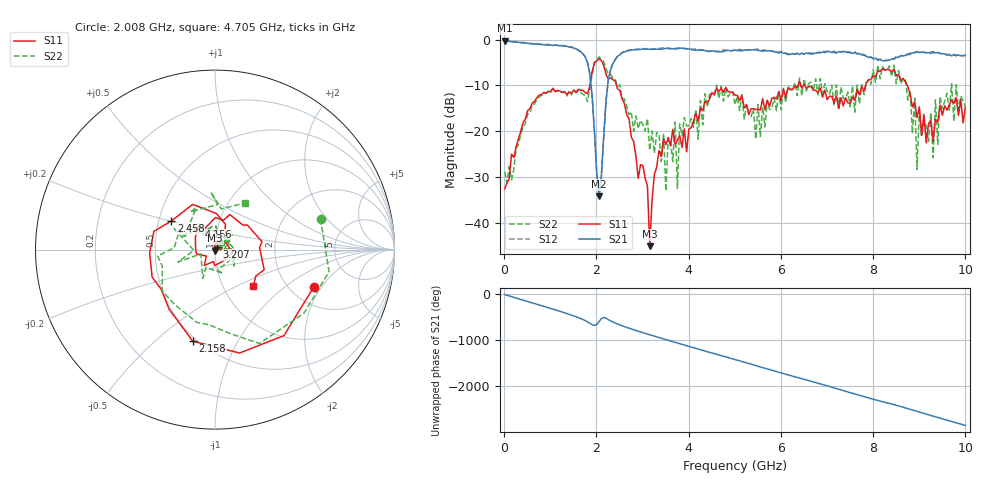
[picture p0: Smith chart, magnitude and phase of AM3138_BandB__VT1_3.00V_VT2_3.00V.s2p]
! Date/Time: Tue, Nov 13, 2018 4:39 PM
! Network Analyzer: Agilent Technologies E8364B Rev: A.07.50.67
! Sweep from 0.010 to 10.000 GHz, 201 Points, Sweep Type: LIN
! Power Supply: 3.001 V, 0.000 A
# Hz S DB R 50
!freq MagS11 AngS11 MagS21 AngS21 MagS12 AngS12 MagS22 AngS22
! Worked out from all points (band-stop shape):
!   201 points, 10 MHz to 10 GHz, reference 50 ohm
!   highest |S21| = -0.23 dB at 10 MHz (marker M1); lowest = -34.1 dB at 2.058 GHz (marker M2)
!   |S21| within 3 dB of the highest: start of sweep to 1.715 GHz; 2.521 GHz to 6.142 GHz (3.621 GHz wide, 83.6 % of centre)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
!   lowest |S11| = -45.0 dB at 3.157 GHz (marker M3), VSWR 1.01, Z = 50 - j0.564 ohm
!   |S11| at or under -10 dB: start of sweep to 1.859 GHz; 2.437 GHz to 6.369 GHz (3.932 GHz wide, 89.3 % of centre); 6.515 GHz to 7.836 GHz (1.321 GHz wide, 18.4 % of centre)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
!   |S22| runs from -33.0 to -3.8 dB; largest |S21 - S12| = 0.029
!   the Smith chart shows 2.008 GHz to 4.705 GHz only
!   S11 on the Smith chart (normalised r, x): 2.008 GHz: 2.64, -1.70; 2.158 GHz: 0.48, -0.67; 2.458 GHz: 0.58, +0.20; 3.207 GHz: 1.02, +0.03; 4.156 GHz: 0.81, +0.21; 4.705 GHz: 1.38, -0.62
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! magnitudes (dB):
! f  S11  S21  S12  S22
! 10 MHz  -32.5  -0.2  -0.2  -28.7
! 1.708 GHz  -11.1  -3.1  -3.0  -11.9
! 2.008 GHz  -4.6  -29.2  -29.0  -4.3
! 2.058 GHz  -4.2  -34.1  -34.3  -3.8
! 2.158 GHz  -5.6  -21.3  -21.3  -4.7
! 2.458 GHz  -10.7  -3.7  -3.6  -10.3
! 3.157 GHz  -45.0  -2.1  -2.1  -24.1
! 3.207 GHz  -34.8  -2.1  -2.1  -19.9
! 3.357 GHz  -24.2  -2.1  -1.9  -20.6
! 3.507 GHz  -22.8  -1.9  -1.9  -33.0
! 3.706 GHz  -22.8  -2.1  -1.9  -17.9
! 3.756 GHz  -21.9  -2.0  -1.9  -32.4
! 3.806 GHz  -20.9  -1.9  -1.8  -18.4
! 4.156 GHz  -16.1  -2.3  -2.1  -15.2
! 4.705 GHz  -10.6  -2.7  -2.5  -10.2
! 5.005 GHz  -12.1  -2.3  -2.2  -14.2
! 6.703 GHz  -11.0  -3.1  -2.9  -11.2
! 8.352 GHz  -6.6  -4.5  -4.4  -5.7
! 8.901 GHz  -13.5  -2.9  -2.8  -12.8
! 8.951 GHz  -17.0  -2.7  -2.6  -28.3
! 9.001 GHz  -14.7  -2.8  -2.8  -15.3
! 10 GHz  -14.7  -3.5  -3.4  -14.7
